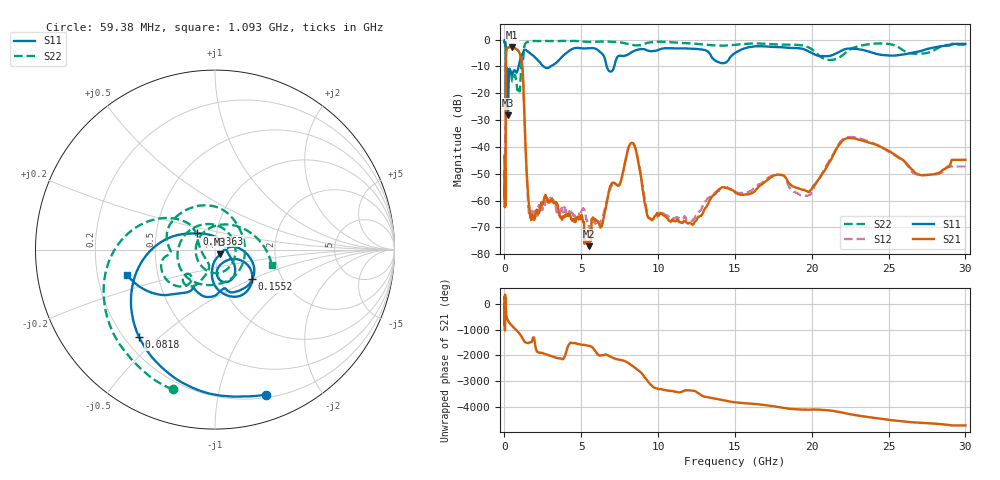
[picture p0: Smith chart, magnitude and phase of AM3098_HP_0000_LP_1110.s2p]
! Date/Time: Thu, Feb 28, 2019 8:31 AM
! Network Analyzer: Agilent Technologies E8364B Rev: A.07.50.67
! Sweep from 0.010 to 30.000 GHz, 1601 Points, Sweep Type: LOG
! Power Supply: 5.022 V, 0.002 A
# Hz S DB R 50
!freq MagS11 AngS11 MagS21 AngS21 MagS12 AngS12 MagS22 AngS22
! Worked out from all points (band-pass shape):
!   1601 points, 10 MHz to 30 GHz, reference 50 ohm
!   highest |S21| = -2.78 dB at 495.6 MHz (marker M1); lowest = -77.0 dB at 5.473 GHz (marker M2)
!   |S21| within 3 dB of the highest: 104.8 MHz to 1.028 GHz (923.4 MHz wide, 163 % of centre)
!   lowest |S11| = -28.3 dB at 231.6 MHz (marker M3), VSWR 1.08, Z = 52.8 - j2.84 ohm
!   |S11| at or under -10 dB: 90.38 MHz to 922.3 MHz (832 MHz wide, 164 % of centre); 2.534 GHz to 2.998 GHz (464.2 MHz wide, 16.8 % of centre); 6.654 GHz to 7.147 GHz (493.3 MHz wide, 7.15 % of centre)
!   |S22| runs from -22.9 to -0.5 dB; largest |S21 - S12| = 0.012
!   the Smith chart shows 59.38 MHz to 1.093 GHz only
!   S11 on the Smith chart (normalised r, x): 59.38 MHz: 0.23, -1.39; 81.8 MHz: 0.26, -0.43; 93.63 MHz: 0.80, +0.15; 155.2 MHz: 1.42, -0.50; 1.093 GHz: 0.33, -0.13
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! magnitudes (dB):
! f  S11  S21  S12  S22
! 10 MHz  -0.3  -43.2  -44.6  -0.6
! 38.04 MHz  -0.5  -60.6  -59.5  -1.0
! 59.38 MHz  -1.3  -51.7  -50.7  -1.8
! 71.46 MHz  -2.0  -53.0  -50.4  -2.5
! 81.8 MHz  -3.8  -32.7  -32.7  -4.2
! 93.63 MHz  -17.3  -11.3  -11.3  -21.1
! 144.7 MHz  -14.3  -3.5  -3.4  -12.7
! 155.2 MHz  -11.6  -3.4  -3.4  -11.0
! 231.6 MHz  -28.3  -2.9  -2.9  -12.0
! 495.6 MHz  -13.1  -2.8  -2.8  -15.3
! 550.5 MHz  -12.5  -3.0  -2.9  -15.1
! 1.093 GHz  -5.9  -7.4  -7.4  -9.7
! 1.567 GHz  -4.6  -60.0  -63.0  -0.8
! 2.084 GHz  -7.1  -63.7  -65.3  -0.5
! 5.473 GHz  -3.3  -77.0  -68.9  -0.8
! 7.926 GHz  -5.9  -43.8  -43.7  -1.5
! 8.501 GHz  -4.1  -40.2  -40.1  -2.2
! 9.538 GHz  -4.4  -67.0  -66.9  -1.0
! 11.83 GHz  -3.3  -68.1  -67.0  -1.4
! 19.61 GHz  -3.9  -56.3  -58.2  -2.5
! 22.67 GHz  -3.4  -36.8  -36.3  -3.2
! 30 GHz  -1.6  -44.8  -47.3  -1.9
